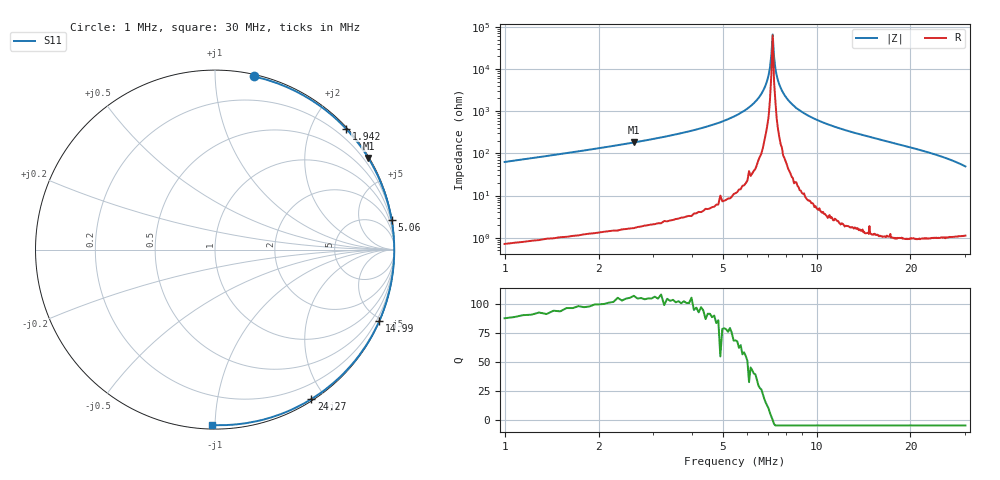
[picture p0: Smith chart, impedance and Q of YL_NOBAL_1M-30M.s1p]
!File
# Hz S RI R 50
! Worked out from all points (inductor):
!   401 points, 1 MHz to 30 MHz, reference 50 ohm
!   read as one part to ground: L = 9.72 uH near 1.145 MHz
!   highest Q = 105 at 2.595 MHz (marker M1), where L = 11.1 uH
!   self-resonance near 7.162 MHz
!   S11 on the Smith chart (normalised r, x): 1 MHz: 0.01, +1.25; 1.942 MHz: 0.03, +2.56; 5.06 MHz: 0, +12; 14.99 MHz: 0.02, -4.79; 24.27 MHz: 0.02, -1.83; 30 MHz: 0.02, -0.98
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1000000  0.2184 0.9645
1145000  0.346 0.9272
1290000  0.4502 0.8822
1507500  0.5713 0.8101
1725000  0.6617 0.7396
1942500  0.7297 0.6737
2232500  0.7965 0.5948
2595000  0.8546 0.51
3030000  0.901 0.4245
3537500  0.9358 0.3427
4045000  0.9585 0.2748
4625000  0.9754 0.2093
5060000  0.9839 0.1663
6437500  0.997 0.054
8250000  0.9967 -0.0625
1.1875e7  0.9663 -0.2519
1.49925e7  0.9145 -0.3995
1.55e7  0.9035 -0.4234
1.74575e7  0.8536 -0.5154
1.9125e7  0.7995 -0.5944
2.101e7  0.7228 -0.6838
2.275e7  0.6333 -0.765
2.42725e7  0.537 -0.8327
2.536e7  0.4567 -0.8774
2.6375e7  0.3716 -0.9147
2.826e7  0.1859 -0.9651
2.92025e7  0.0792 -0.9768
3e7  -0.0183 -0.9772
